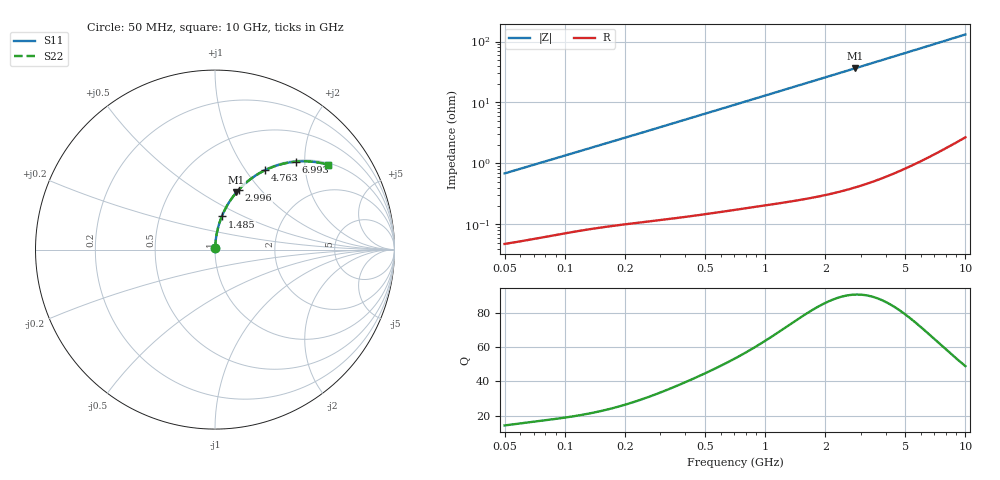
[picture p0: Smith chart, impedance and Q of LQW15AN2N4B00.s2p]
!Murata Part Number: LQW15AN2N4B00
!These Parameters are Measured in Series Mode Connection
!  o--[Z]--o
!Port1  Port2
!  o-------o
!Freq. Start=50[MHz] Stop=10[GHz], 401[Steps]
# Hz S RI R 50
!Freq.(Hz)	S 11(Real)	S 11(Imag)	S 21(Real)	S 21(Imag)	S 12(Real)	S 12(Imag)	S 22(Real)	S 22(Imag)
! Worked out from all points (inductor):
!   401 points, 50 MHz to 10 GHz, reference 50 ohm
!   read as one part in series: L = 2.16 nH near 51.34 MHz
!   highest Q = 90.5 at 2.804 GHz (marker M1), where L = 2.06 nH
!   S11 on the Smith chart (normalised r, x): 50 MHz: 1.00, +0.01; 1.485 GHz: 1.01, +0.38; 2.996 GHz: 1.01, +0.78; 4.763 GHz: 1.02, +1.23; 6.993 GHz: 1.03, +1.82; 10 GHz: 1.05, +2.61
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5e7  0.000523 0.00682  0.9995 -0.00682  0.9995 -0.00682  0.000523 0.00682
5.134228e7  0.000532 0.007  0.9995 -0.007  0.9995 -0.007  0.000532 0.007
1.214486e8  0.00105 0.0162  0.9989 -0.0162  0.9989 -0.0162  0.00105 0.0162
1.956524e8  0.00166 0.0258  0.9983 -0.0258  0.9983 -0.0258  0.00166 0.0258
2.949953e8  0.00266 0.0386  0.9973 -0.0386  0.9973 -0.0386  0.00266 0.0386
4.689809e8  0.00514 0.0608  0.9949 -0.0608  0.9949 -0.0608  0.00514 0.0608
7.071068e8  0.0101 0.0909  0.9899 -0.0909  0.9899 -0.0909  0.0101 0.0909
1.038268e9  0.0198 0.1317  0.9802 -0.1317  0.9802 -0.1317  0.0198 0.1317
1.249815e9  0.0277 0.1571  0.9723 -0.1571  0.9723 -0.1571  0.0277 0.1571
1.484667e9  0.0379 0.1845  0.9621 -0.1845  0.9621 -0.1845  0.0379 0.1845
1.717543e9  0.0494 0.2107  0.9506 -0.2107  0.9506 -0.2107  0.0494 0.2107
2.23851e9  0.0799 0.2656  0.9201 -0.2656  0.9201 -0.2656  0.0799 0.2656
2.803837e9  0.119 0.3183  0.881 -0.3183  0.881 -0.3183  0.119 0.3183
2.99582e9  0.1333 0.3344  0.8667 -0.3344  0.8667 -0.3344  0.1333 0.3344
3.558764e9  0.1777 0.3767  0.8223 -0.3767  0.8223 -0.3767  0.1777 0.3767
4.171863e9  0.2285 0.414  0.7715 -0.414  0.7715 -0.414  0.2285 0.414
4.762728e9  0.2782 0.4419  0.7218 -0.4419  0.7218 -0.4419  0.2782 0.4419
5.809576e9  0.364 0.4743  0.636 -0.4743  0.636 -0.4743  0.364 0.4743
6.993273e9  0.453 0.4901  0.547 -0.4901  0.547 -0.4901  0.453 0.4901
8.307378e9  0.5387 0.4898  0.4613 -0.4898  0.4613 -0.4898  0.5387 0.4898
9.738562e9  0.616 0.4764  0.384 -0.4764  0.384 -0.4764  0.616 0.4764
1e10  0.6285 0.4731  0.3715 -0.4731  0.3715 -0.4731  0.6285 0.4731
